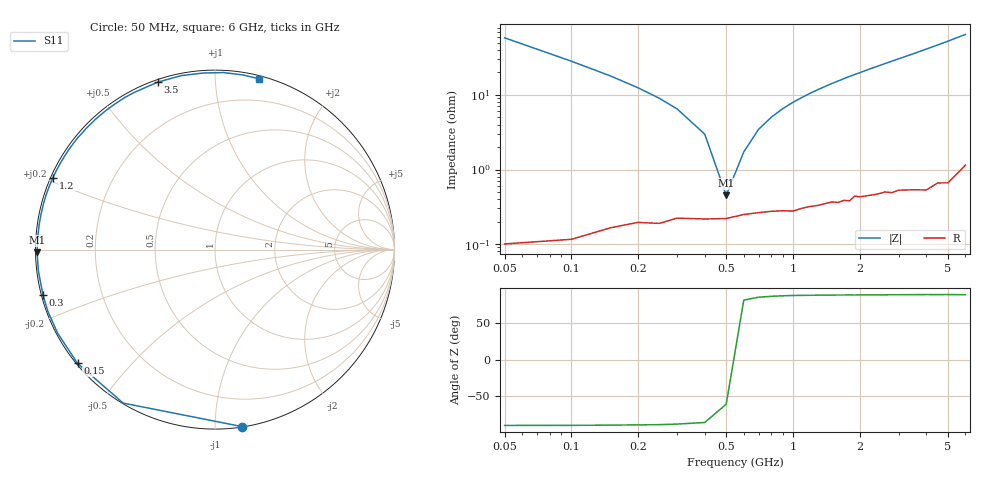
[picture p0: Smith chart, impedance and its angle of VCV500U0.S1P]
! Infineon Technologies  Discrete & RF Semiconductors
! BBY 56-03
! Si Tuning Diode in SOD323
! VR = 0.5 V
! S-Parameters:  June  1999
# GHz  S  MA  R  50
!  f  S11
! GHz  MAG  ANG
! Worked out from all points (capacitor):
!   34 points, 50 MHz to 6 GHz, reference 50 ohm
!   read as one part to ground: C = 54.1 pF near 50 MHz
!   lowest |Z| = 450 mohm at 500 MHz (marker M1)
!   series resonance near 518.7 MHz, so ESL is about 1.7 nH
!   S11 on the Smith chart (normalised r, x): 50 MHz: 0.00, -1.17; 150 MHz: 0.00, -0.36; 300 MHz: 0.00, -0.13; 1.2 GHz: 0.01, +0.21; 3.5 GHz: 0.01, +0.71; 6 GHz: 0.02, +1.29
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0.05  0.9983 -81.2
0.1  0.9965 -120.9
0.15  0.9942 -140.4
0.2  0.9927 -152.0
0.25  0.9927 -159.6
0.3  0.9913 -165.2
0.4  0.9914 -173.2
0.5  0.9912 -179.1
0.6  0.9901 176.1
0.7  0.9895 172.1
0.8  0.9892 168.5
1  0.9893 161.9
1.2  0.9878 156.1
1.4  0.987 150.8
1.6  0.9869 145.8
1.8  0.9866 141.0
1.9  0.9847 138.8
2.2  0.9851 132.4
2.4  0.985 128.4
2.6  0.9845 124.5
2.8  0.9853 120.8
3  0.9847 117.2
3.5  0.9859 108.9
4  0.9874 101.0
4.5  0.986 93.8
5  0.9875 87.2
5.5  0.9854 80.9
6  0.983 75.4
